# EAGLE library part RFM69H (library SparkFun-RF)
Hope RF RFM69H ISM Transceiver Module The RFM69H is a transceiver module capable of operation over a wide frequency range, including the 315,433,868 and 915MHz license-free ISM (Industry Scientific and Medical) frequency bands. All major RF communication parameters are programmable and most of them can be dynamically set. The RFM69H offers the unique advantage of programmable narrow-band and wide- band communication modes. The RFM69H is optimized for low power consumption while offering high RF output power and channelized operation.Compliance ETSI and FCC regulations. Datasheet SparkFun Products RFM69HCW Wireless Transceiver - 915MHz (COM-13909) RFM69HCW Wireless Transceiver - 434MHz (COM-13910) SparkFun RFM69 Breakout (915MHz) (WRL-12775) SparkFun RFM69 Breakout (434MHz) (WRL-12823)
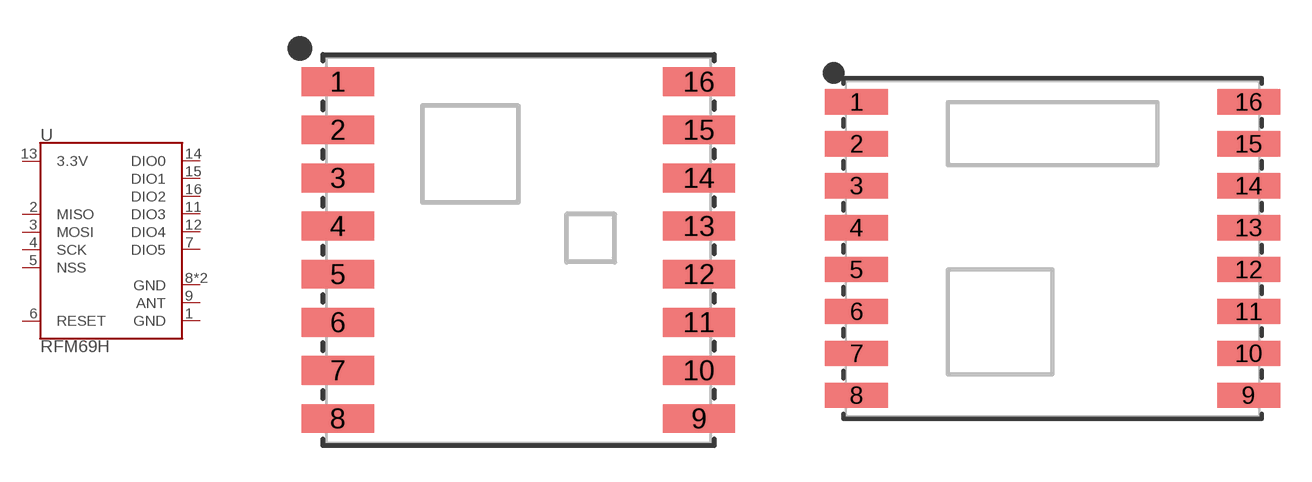
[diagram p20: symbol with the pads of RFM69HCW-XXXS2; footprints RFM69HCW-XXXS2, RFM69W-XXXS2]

Designator prefix U

## RFM69HCW-915 (PROD_ID: IC-11997; VALUE: 915MHz)  [RFM69HCW-XXXS2]
1  GND  pwr
2  MISO
3  MOSI  in
4  SCK  in
5  NSS  in
6  RESET  in
7  DIO5
8  GND  pwr
9  ANT  pas
10  GND  pwr
11  DIO3
12  DIO4
13  3.3V  pwr
14  DIO0
15  DIO1
16  DIO2

## RFM69HW  [RFM69W-XXXS2]
1  RESET  in
2  DIO0
3  DIO1
4  DIO2
5  DIO3
6  DIO4
7  DIO5
8  3.3V  pwr
9  GND  pwr
10  ANT  pas
11  GND  pwr
12  SCK  in
13  MISO
14  MOSI  in
15  NSS  in

## RFM69HCW-433 (PROD_ID: IC-12053; VALUE: 433MHz)  [RFM69HCW-XXXS2]
Pads as for RFM69HCW-XXXS2

## Footprint RFM69HCW-XXXS2 (pad centres in mm)
Hope RF RFM69HCW RF Transciever Datasheet
smd 3 x 1.2: 1 -7.5,7; 2 -7.5,5; 3 -7.5,3; 4 -7.5,1; 5 -7.5,-1; 6 -7.5,-3; 7 -7.5,-5; 8 -7.5,-7; 9 7.5,-7; 10 7.5,-5; 11 7.5,-3; 12 7.5,-1; 13 7.5,1; 14 7.5,3; 15 7.5,5; 16 7.5,7

## Footprint RFM69W-XXXS2 (pad centres in mm)
Hope RF RFM69HW RF Transceiver Datasheet
smd 3 x 1.2: 1 -9.35,7; 2 -9.35,5; 3 -9.35,3; 4 -9.35,1; 5 -9.35,-1; 6 -9.35,-3; 7 -9.35,-5; 8 -9.35,-7; 9 9.35,-7; 10 9.35,-5; 11 9.35,-3; 12 9.35,-1; 13 9.35,1; 14 9.35,3; 15 9.35,5; 16 9.35,7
